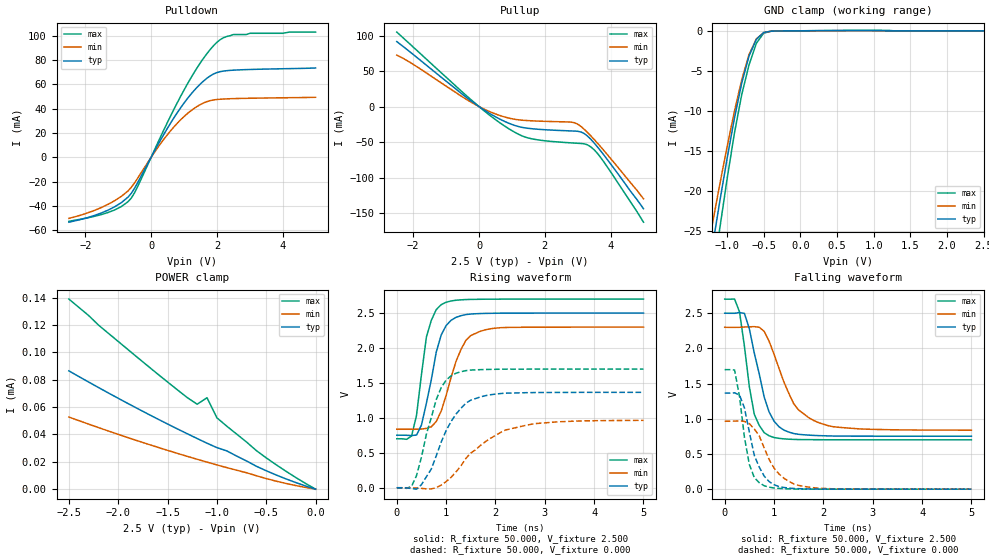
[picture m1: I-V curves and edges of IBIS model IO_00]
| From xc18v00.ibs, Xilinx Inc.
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|   Model IO_00
[Model]   IO_00
Model_type   I/O
Polarity   Inverting
Enable   Active-High
Vinl =   0.800V
Vinh =   2.000V
Vmeas =   1.250V
Cref =  50.000pF
Rref =   1.000M
Vref =  0.000V
C_comp   6.700pF   5.700pF   7.600pF
[Temperature Range]   50.000   100.000   0.000
[Voltage Range]   2.500V   2.300V   2.700V
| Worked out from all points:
|   slope of the pulldown table from 0 to 0.375 V, typ, clamps not added: 20.4 ohm
|   slope of the pullup table from 0 to 0.375 V, typ, clamps not added: 33.7 ohm
|   GND clamp passes 1 mA (typ) near -0.59 V on its own axis
|   rising waveform, R_fixture 50.000, V_fixture 2.500: 20-80 % time 320ps typ, 408ps min, 249ps max; typ from 0.752 V to 2.5 V
|   rising waveform, R_fixture 50.000, V_fixture 0.000: 20-80 % time 544ps typ, 897ps min, 394ps max; typ from 0 V to 1.36 V
|   falling waveform, R_fixture 50.000, V_fixture 2.500: 20-80 % time 361ps typ, 541ps min, 246ps max; typ from 2.5 V to 0.752 V
|   falling waveform, R_fixture 50.000, V_fixture 0.000: 20-80 % time 313ps typ, 452ps min, 216ps max; typ from 1.36 V to 0 V
[Pulldown]
| voltage   I(typ)   I(min)   I(max)
-2.5V     -53.3mA    -50.18mA   -52.6mA
-1.3V     -43.29mA   -38.5mA    -45.24mA
-900mV    -37.13mA   -31.98mA   -40.37mA
-600mV    -29.49mA   -24.58mA   -33.4mA
-400mV    -20.36mA   -16.75mA   -23.48mA
300mV     14.82mA    11.72mA    17.61mA
900mV     40.85mA    30.95mA    50.29mA
1.3V      54.75mA    40.1mA     69.38mA
1.6V      62.9mA     44.78mA    81.74mA
2.1V      70.47mA    47.8mA     96.78mA
2.5V      71.69mA    48.3mA     101mA
5V        73.49mA    49.4mA     103mA
[Pullup]
| voltage   I(typ)   I(min)   I(max)
-2.5V     91.64mA    72.63mA    105mA
-200mV    6.597mA    5.069mA    7.944mA
400mV     -11.81mA   -8.597mA   -14.94mA
900mV     -23.39mA   -16.16mA   -31.1mA
1.3V      -29.26mA   -19.18mA   -41.18mA
1.6V      -31.21mA   -20.09mA   -45.4mA
2.8V      -34.35mA   -21.93mA   -51.18mA
3V        -34.86mA   -24.83mA   -51.75mA
3.3V      -41.63mA   -36.61mA   -54.02mA
3.6V      -56.87mA   -51.52mA   -65.98mA
4V        -80.78mA   -73.13mA   -91.93mA
5V        -144mA     -130mA     -163mA
[GND_clamp]
| voltage   I(typ)   I(min)   I(max)
-2.5V     -106mA     -95.22mA   -120mA
-1.2V     -26.97mA   -24.12mA   -31.21mA
-1.1V     -21.35mA   -19.21mA   -24.73mA
-1V       -15.97mA   -14.5mA    -18.53mA
-900mV    -10.95mA   -10.08mA   -12.81mA
-800mV    -6.536mA   -6.124mA   -7.972mA
-700mV    -3.151mA   -2.957mA   -4.247mA
-600mV    -1.058mA   -1.006mA   -1.557mA
-500mV    -212uA     -231uA     -287uA
-400mV    -45.28uA   -47.34uA   -59.63uA
100mV     5.458uA    3.158uA    9.403uA
2.5V      1.486nA    2.623uA    -7.463uA
[POWER_clamp]
| voltage   I(typ)   I(min)   I(max)
-2.5V     86.5uA     52.74uA    139uA
-2.3V     78.34uA    47.57uA    127uA
-2.2V     74.33uA    45.03uA    120uA
-1.7V     55.02uA    32.94uA    90.07uA
-1.3V     40.51uA    23.99uA    66.94uA
-1.2V     37.02uA    21.86uA    62.11uA
-1.1V     33.6uA     19.77uA    66.85uA
-1V       30.39uA    17.73uA    52.18uA
-900mV    28uA       15.75uA    46.06uA
-500mV    13.46uA    7.741uA    22.89uA
-200mV    4.817uA    2.623uA    8.493uA
0V        1.483nA    6.217nA    302pA
[Ramp]
| variable   typ   min   max
dV/dt_r   0.819/0.540n   0.578/0.904n   1.019/0.360n
dV/dt_f   1.049/0.330n   0.877/0.563n   1.199/0.228n
R_load = 50.000
[Rising Waveform]
R_fixture = 50.000
V_fixture = 2.500
V_fixture_min = 2.300
V_fixture_max = 2.700
L_fixture = 0.000H
C_fixture = 0.000F
| time   V(typ)   V(min)   V(max)
0s        752mV      837mV      701mV
300ps     747mV      837mV      741mV
400ps     754mV      837mV      1.035V
500ps     897mV      840mV      1.618V
600ps     1.209V     849mV      2.156V
700ps     1.547V     872mV      2.396V
900ps     2.186V     1.096V     2.62V
1.3ns     2.462V     1.976V     2.689V
1.7ns     2.493V     2.241V     2.697V
5ns       2.499V     2.299V     2.7V
[Rising Waveform]
R_fixture = 50.000
V_fixture = 0.000
V_fixture_min = 0.000
V_fixture_max = 0.000
L_fixture = 0.000H
C_fixture = 0.000F
| time   V(typ)   V(min)   V(max)
0s        0V         0V         0V
300ps     -11.79mV   -884uV     20.59mV
500ps     44.89mV    -9.011mV   438mV
700ps     268mV      -16.52mV   1.007V
900ps     654mV      38.09mV    1.433V
1.2ns     1.053V     225mV      1.639V
1.5ns     1.254V     496mV      1.684V
2.2ns     1.353V     825mV      1.697V
3.2ns     1.364V     940mV      1.698V
5ns       1.365V     964mV      1.698V
[Falling Waveform]
R_fixture = 50.000
V_fixture = 2.500
V_fixture_min = 2.300
V_fixture_max = 2.700
L_fixture = 0.000H
C_fixture = 0.000F
| time   V(typ)   V(min)   V(max)
0s        2.5V       2.3V       2.7V
200ps     2.499V     2.299V     2.701V
300ps     2.509V     2.3V       2.52V
400ps     2.497V     2.304V     2.029V
500ps     2.278V     2.307V     1.454V
600ps     1.933V     2.309V     1.063V
900ps     1.097V     2.102V     758mV
1.4ns     790mV      1.212V     707mV
1.9ns     761mV      946mV      703mV
5ns       752mV      838mV      701mV
[Falling Waveform]
R_fixture = 50.000
V_fixture = 0.000
V_fixture_min = 0.000
V_fixture_max = 0.000
L_fixture = 0.000H
C_fixture = 0.000F
| time   V(typ)   V(min)   V(max)
0s        1.365V     965mV      1.698V
200ps     1.369V     967mV      1.693V
300ps     1.338V     970mV      1.318V
400ps     1.155V     963mV      737mV
500ps     810mV      930mV      350mV
600ps     480mV      854mV      165mV
800ps     186mV      587mV      48.87mV
1.1ns     37.06mV    216mV      10.58mV
1.5ns     6.726mV    52.91mV    1.766mV
5ns       9.319uV    61.34uV    0V
